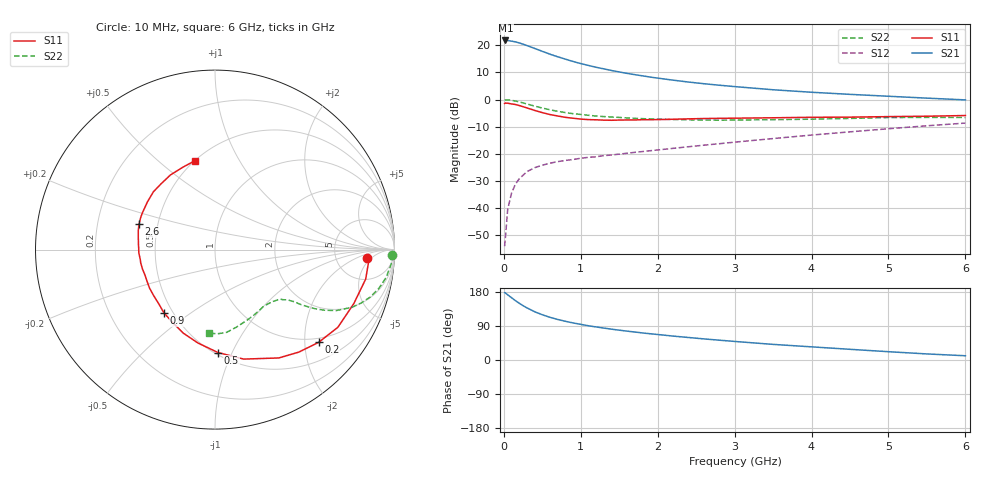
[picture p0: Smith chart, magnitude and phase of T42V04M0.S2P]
! Infineon Technologies  Discrete & RF Semiconductors
! BFR182T
! Si NPN RF Bipolar Junction Transistor in SC75
! VCE = 2 V  IC = 4 mA
! Common Emitter S-Parameters:  October  1999
# GHz  S  MA  R  50
!  f  S11  S21  S12  S22
! GHz  MAG  ANG  MAG  ANG  MAG  ANG  MAG  ANG
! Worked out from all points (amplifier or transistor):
!   36 points, 10 MHz to 6 GHz, reference 50 ohm
!   highest |S21| = 21.7 dB at 20 MHz (marker M1)
!   |S21| within 3 dB of that: start of sweep to 407.1 MHz
!   unconditionally stable (mu >= 1): 1.509 GHz to 4.112 GHz
!   at 250 MHz: K = 0.23, MSG = 24.1 dB, |S12| = -27.9 dB
!   at 1.4 GHz: K = 0.98, MSG = 15.6 dB, |S12| = -20.4 dB
!   at 6 GHz: K = 0.84, MSG = 4.3 dB, |S12| = -8.7 dB
!   S11 on the Smith chart (normalised r, x): 10 MHz: 11, -4; 200 MHz: 0.90, -2.32; 500 MHz: 0.52, -0.89; 900 MHz: 0.45, -0.40; 2.6 GHz: 0.39, +0.14; 6 GHz: 0.50, +0.67
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0.01  0.847 -3.3  12.18 177.8  0.002 81.8  0.9861 -1.7
0.02  0.8609 -3.1  12.21 177.0  0.0028 97.3  0.985 -1.9
0.05  0.8554 -11.1  12.18 172.0  0.0095 87.0  0.985 -4.7
0.1  0.8298 -21.3  11.86 164.4  0.0189 79.8  0.9664 -9.2
0.15  0.8099 -32.3  11.51 156.7  0.0276 73.5  0.9375 -13.4
0.2  0.7749 -41.8  11.02 149.8  0.0348 70.7  0.9047 -17.0
0.25  0.7379 -50.7  10.43 143.4  0.0404 65.8  0.8664 -20.1
0.3  0.7006 -59.5  9.84 137.6  0.047 62.4  0.8294 -22.8
0.4  0.6307 -75.3  8.724 127.4  0.0556 56.5  0.7561 -26.7
0.5  0.5739 -88.3  7.696 119.4  0.0618 53.0  0.6965 -29.0
0.6  0.5289 -100.4  6.825 112.6  0.0673 51.4  0.6468 -30.6
0.7  0.4976 -110.9  6.121 107.0  0.0719 50.2  0.6069 -31.6
0.9  0.4528 -129.0  5.01 97.8  0.0787 49.1  0.5484 -33.0
1.1  0.4269 -143.5  4.236 90.3  0.0863 49.4  0.5125 -34.0
1.3  0.4174 -155.6  3.665 84.2  0.0928 50.4  0.4853 -35.2
1.6  0.4204 -169.8  3.03 76.2  0.1026 52.3  0.458 -37.1
2.2  0.4328 170.9  2.27 63.1  0.1262 56.4  0.4294 -43.2
2.6  0.4465 161.4  1.953 55.7  0.1444 58.3  0.4188 -48.0
3.5  0.461 144.6  1.512 41.2  0.1912 60.0  0.4257 -60.2
4.5  0.474 129.3  1.244 28.2  0.2542 58.4  0.4488 -74.8
5.5  0.4927 111.4  1.06 16.0  0.3285 54.1  0.4693 -88.3
6  0.5073 102.8  0.984 11.2  0.3686 50.8  0.4668 -94.2
